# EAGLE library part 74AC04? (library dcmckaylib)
Inverter
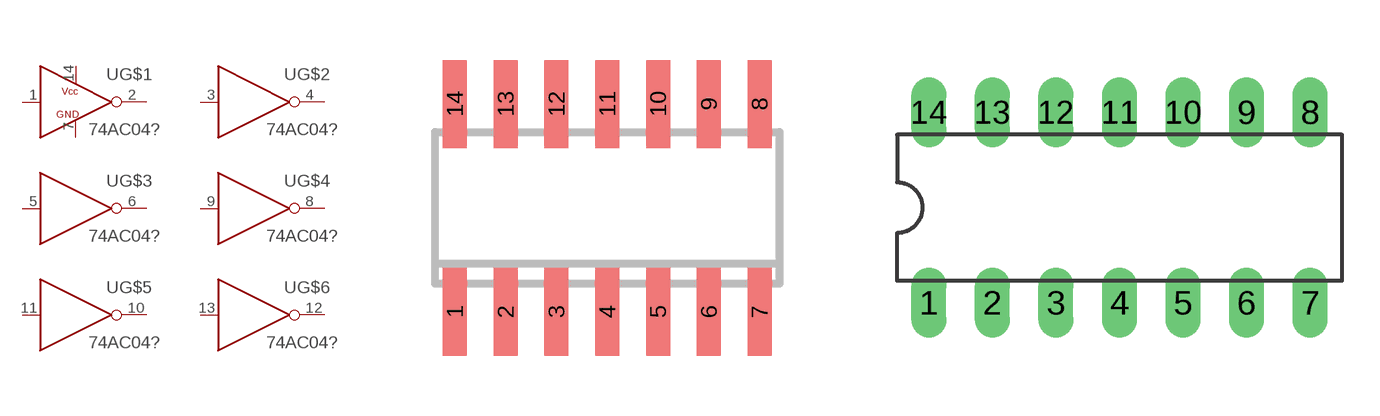
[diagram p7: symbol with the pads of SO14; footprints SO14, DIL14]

Designator prefix -; gates G$1=INVERTER2 G$2=INVERTER G$3=INVERTER G$4=INVERTER G$5=INVERTER G$6=INVERTER

## 74AC04SC  [SO14]
1  G$1:IN  in
2  G$1:OUT  out
3  G$2:IN  in
4  G$2:OUT  out
5  G$3:IN  in
6  G$3:OUT  out
7  G$1:GND
8  G$4:OUT  out
9  G$4:IN  in
10  G$5:OUT  out
11  G$5:IN  in
12  G$6:OUT  out
13  G$6:IN  in
14  G$1:VCC

## 74AC04PC  [DIL14]
Pads as for SO14

## Footprint SO14 (pad centres in mm)
Small Outline Package 14
smd 0.6 x 2.2: 1 -3.81,-2.6; 2 -2.54,-2.6; 3 -1.27,-2.6; 4 0,-2.6; 5 1.27,-2.6; 6 2.54,-2.6; 7 3.81,-2.6; 8 3.81,2.6; 9 2.54,2.6; 10 1.27,2.6; 11 0,2.6; 12 -1.27,2.6; 13 -2.54,2.6; 14 -3.81,2.6

## Footprint DIL14 (pad centres in mm)
Dual In Line Package
drill 0.889 long: 1 -7.62,-3.81; 2 -5.08,-3.81; 3 -2.54,-3.81; 4 0,-3.81; 5 2.54,-3.81; 6 5.08,-3.81; 7 7.62,-3.81; 8 7.62,3.81; 9 5.08,3.81; 10 2.54,3.81; 11 0,3.81; 12 -2.54,3.81; 13 -5.08,3.81; 14 -7.62,3.81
